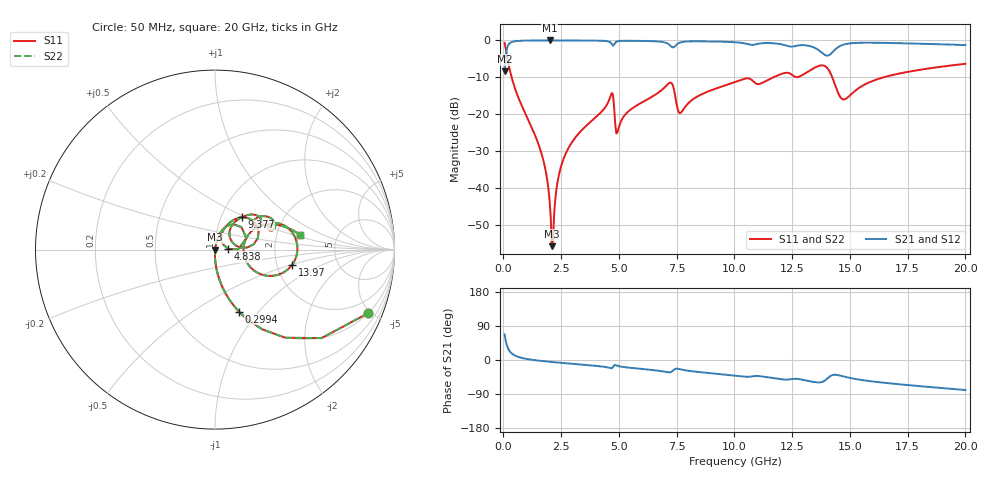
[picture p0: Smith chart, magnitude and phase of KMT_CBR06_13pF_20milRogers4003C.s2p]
! Data measured by Modelithics Inc. support@modelithics.com 813-866-6335
! KEMET CBR0603 13pF, Pad Width= 0.851mm, Pad Length= 0.64mm, Pad Gap= 0.62mm, 20mil Rogers 4003C substrate Data, January 2022
# hz S ma R 50
! 2 Port Network Data from SP1.SP block
! freq  magS11  angS11  magS21  angS21  magS12  angS12  magS22  angS22
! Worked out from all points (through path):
!   401 points, 50 MHz to 20 GHz, reference 50 ohm
!   highest |S21| = -0.01 dB at 1.995 GHz (marker M1); lowest = -8.4 dB at 50 MHz (marker M2)
!   group delay of S21, straight-line fit = 11.4 ps
!   lowest |S11| = -55.7 dB at 2.095 GHz (marker M3), VSWR 1.00, Z = 50.1 - j0.126 ohm
!   |S11| at or under -10 dB: 354.4 MHz to 11.69 GHz (11.33 GHz wide, 188 % of centre); 14.24 GHz to 16.45 GHz (2.217 GHz wide, 14.5 % of centre)
!   |S22| runs from -55.7 to -0.7 dB; largest |S21 - S12| = 0
!   S11 on the Smith chart (normalised r, x): 50 MHz: 0.99, -4.83; 299.4 MHz: 0.99, -0.79; 4.838 GHz: 1.16, +0.01; 9.377 GHz: 1.25, +0.47; 13.97 GHz: 2.44, -0.51; 20 GHz: 2.73, +0.57
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5e7  0.9245 -22.5  0.3808 67.5  0.3808 67.5  0.9245 -22.5
2.99375e8  0.3694 -69.0  0.9287 20.9  0.9287 20.9  0.3694 -69.0
1.646e9  0.02952 -90.5  0.9985 -2.5  0.9985 -2.5  0.02952 -90.5
1.8455e9  0.01604 -89.9  0.9987 -3.8  0.9987 -3.8  0.01604 -89.9
1.995125e9  0.006967 -85.3  0.9988 -4.7  0.9988 -4.7  0.006967 -85.3
2.094875e9  0.001639 -50.0  0.9988 -5.3  0.9988 -5.3  0.001639 -50.0
2.194625e9  0.004488 68.7  0.9987 -5.9  0.9987 -5.9  0.004488 68.7
2.54375e9  0.02213 78.9  0.9984 -7.8  0.9984 -7.8  0.02213 78.9
3.391625e9  0.061 76.3  0.9963 -12.2  0.9963 -12.2  0.061 76.3
4.6385e9  0.1768 52.4  0.9367 -21.6  0.9367 -21.6  0.1768 52.4
4.838e9  0.07459 3.1  0.9282 -13.6  0.9282 -13.6  0.07459 3.1
4.987625e9  0.06518 56.9  0.9791 -16.3  0.9791 -16.3  0.06518 56.9
6.73325e9  0.199 57.3  0.9656 -28.6  0.9656 -28.6  0.199 57.3
7.232e9  0.2693 30.6  0.8479 -32.3  0.8479 -32.3  0.2693 30.6
7.680875e9  0.1049 35.7  0.9439 -24.8  0.9439 -24.8  0.1049 35.7
9.376625e9  0.2333 50.4  0.9627 -37.3  0.9627 -37.3  0.2333 50.4
1.0025e10  0.2742 45.2  0.9447 -41.3  0.9447 -41.3  0.2742 45.2
1.336662e10  0.4096 19.0  0.8195 -57.2  0.8195 -57.2  0.4096 19.0
1.396512e10  0.4389 -11.0  0.6261 -52.0  0.6261 -52.0  0.4389 -11.0
1.471325e10  0.159 -1.6  0.8751 -43.2  0.8751 -43.2  0.159 -1.6
1.670825e10  0.3321 25.1  0.9234 -61.5  0.9234 -61.5  0.3321 25.1
2e10  0.4829 9.5  0.8648 -79.3  0.8648 -79.3  0.4829 9.5
